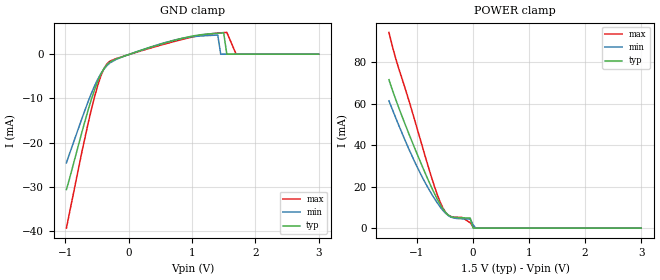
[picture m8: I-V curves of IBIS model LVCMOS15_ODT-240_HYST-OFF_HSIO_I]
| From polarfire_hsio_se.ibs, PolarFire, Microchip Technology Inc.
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|   Model LVCMOS15_ODT-240_HYST-OFF_HSIO_I
[Model]   LVCMOS15_ODT-240_HYST-OFF_HSIO_I
Model_type   Input
Vinl =   0.525
Vinh =   0.975
|   typ   min   max
C_comp_pullup   1.335e-12   1.335e-12   1.380e-12
C_comp_pulldown  1.335e-12   1.335e-12   1.380e-12
[Temperature Range]  25C   100C   -40C
[Voltage Range]  1.5   1.425   1.575
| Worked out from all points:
|   GND clamp passes 1 mA (typ) near -0.18 V on its own axis
|   POWER clamp passes 1 mA (typ) near -0.01 V on its own axis
[GND Clamp]
| Voltage   I(typ)   I(min)   I(max)
-984.4mV  -30.62mA   -24.55mA   -39.33mA
-738.3mV  -17.53mA   -14.48mA   -21.96mA
-541.4mV  -8.093mA   -7.208mA   -9.706mA
-393.7mV  -3.301mA   -3.4mA     -3.312mA
-295.3mV  -1.761mA   -1.953mA   -1.554mA
1.125V    4.376mA    4.101mA    4.247mA
1.406V    4.737mA    4.338mA    4.771mA
1.453V    4.782mA    0A         4.828mA
1.5V      4.826mA    0A         4.882mA
1.549V    0A         0A         4.936mA
1.697V    0A         0A         0A
3V        0A         0A         0A
[POWER Clamp]
| Voltage   I(typ)   I(min)   I(max)
-1.5V     71.65mA    61.45mA    94.5mA
-1.378V   62.05mA    53.19mA    81.78mA
-1.034V   38.16mA    31.63mA    51.52mA
-885.9mV  28.62mA    23.59mA    37.72mA
-689.1mV  16.76mA    14.32mA    20.24mA
-541.4mV  9.477mA    8.704mA    9.945mA
-443mV    6.353mA    6.099mA    6.281mA
-196.9mV  5.004mA    4.515mA    5.168mA
-49.22mV  4.871mA    4.389mA    2.586mA
0V        0A         1.749mA    888.9uA
46.88mV   0A         0A         0A
3V        0A         0A         0A
